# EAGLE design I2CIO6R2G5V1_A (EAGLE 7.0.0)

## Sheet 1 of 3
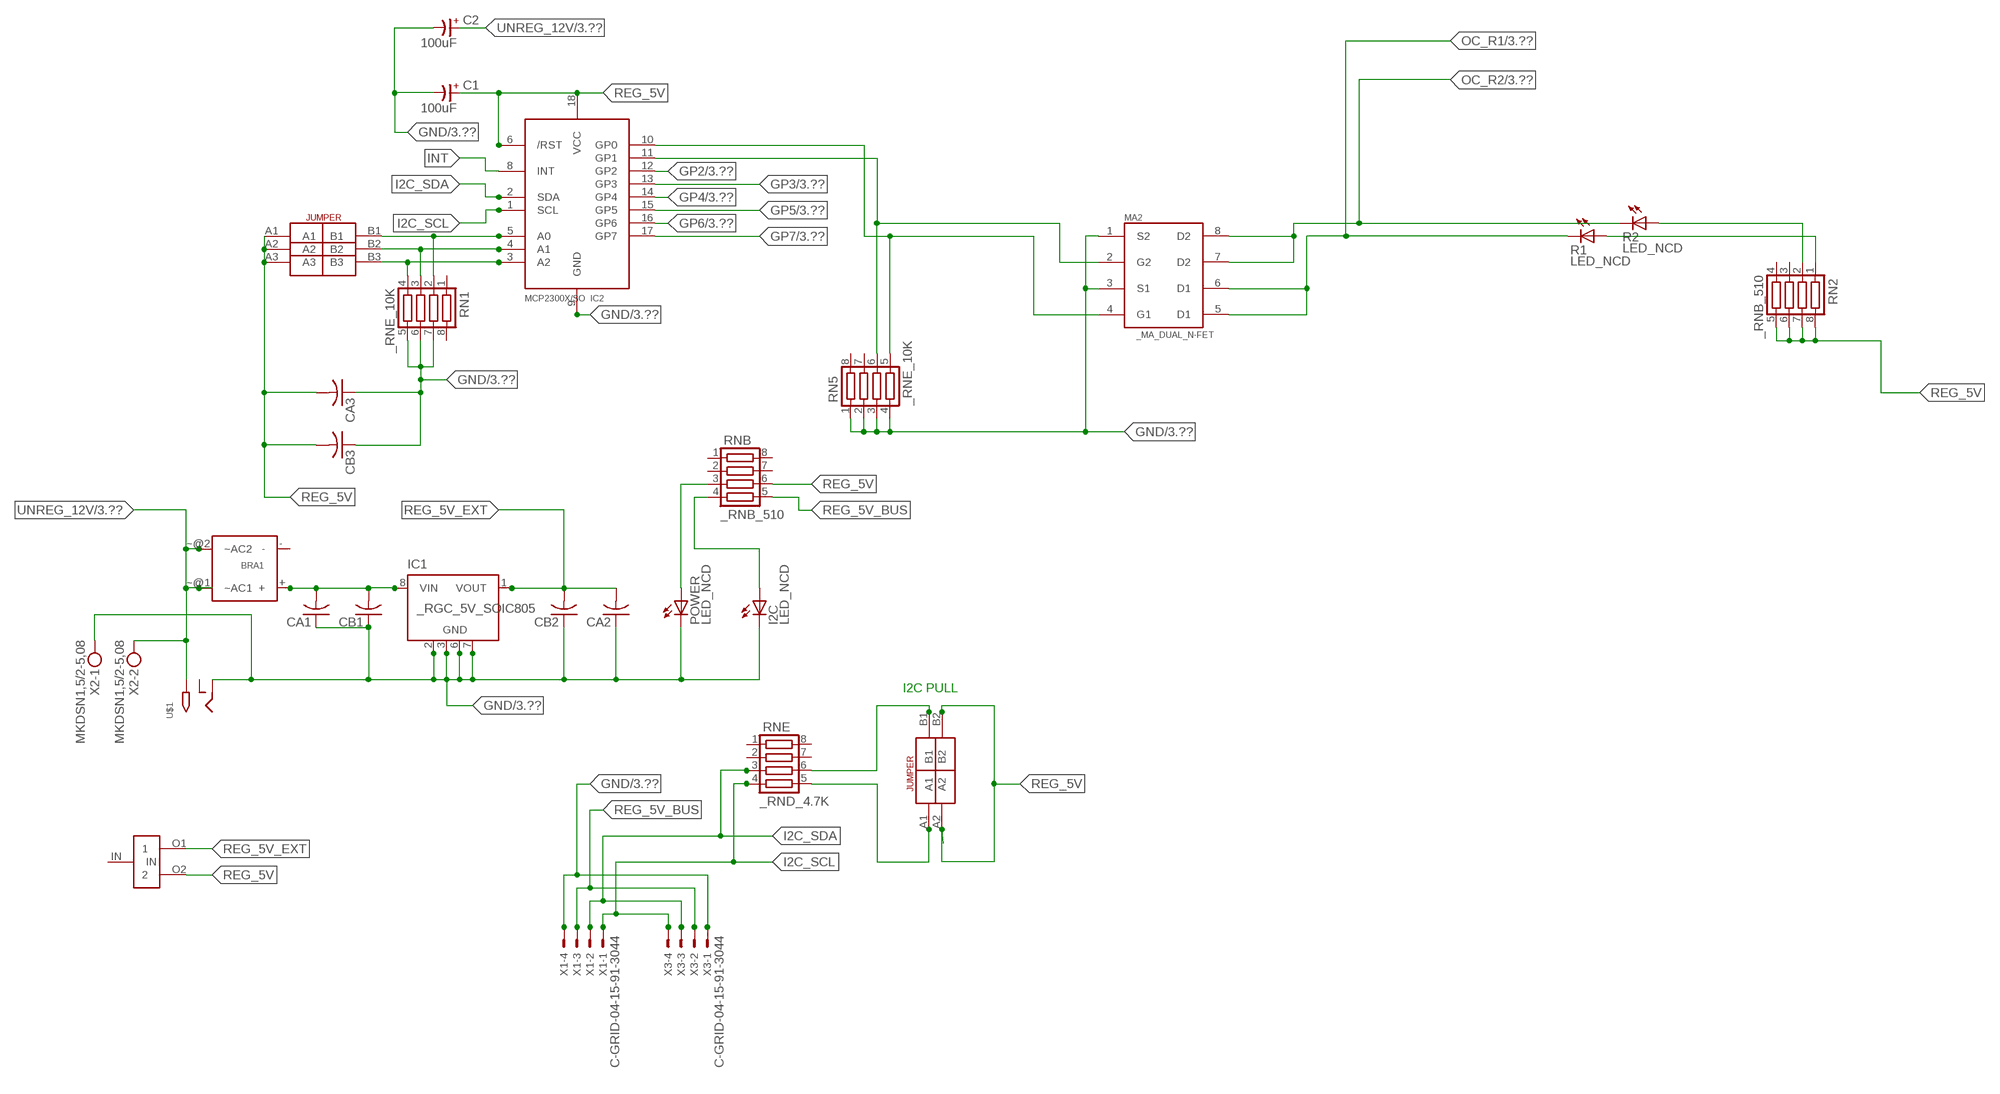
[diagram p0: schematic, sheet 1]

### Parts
BRA1  MB2S_  [MB2S]
C1  100uF  CP-E-025X060  [E-025X060]
C2  100uF  CP-E-025X060  [E-025X060]
CA1  CC1206KRX7R9BB104C1206K  [CC1206KRX7R9BB104]
CA2  CC1206KRX7R9BB104C1206K  [CC1206KRX7R9BB104]
CA3  CC1206KRX7R9BB104C1206K  [CC1206KRX7R9BB104]
CB1  TMK316F106ZL-TC1206K  [TMK316F106ZL-T]
CB2  TMK316F106ZL-TC1206K  [TMK316F106ZL-T]
CB3  TMK316F106ZL-TC1206K  [TMK316F106ZL-T]
I2C  LED_NCD  [CHIPLED_0603]
IC1  _RGC_5V_SOIC805  [_RGC_5V_SOIC8]
IC2  MCP2300X/SO  [SO18W]
MA2  _MA_DUAL_N-FET  [_MA_DUAL_N-FET]
POWER  LED_NCD  [CHIPLED_0603]
R1  LED_NCD  [CHIPLED_0603]
R2  LED_NCD  [CHIPLED_0603]
RN1  _RNE_10K  [RNE]
RN2  _RNB_510  [RNB]
RN5  _RNE_10K  [RNE]
RNB  _RNB_510  [RNB]
RNE  _RND_4.7K  [RND]
U$1  2.1MMJACK  [PJ-102A]
U$3  JUMPER_2X2  [JUMPER_2X2]
U$5  LINK_2  [LINK_2]
U$18  JUMPER_3X2  [JUMPER_3X2]
X1  C-GRID-04-15-91-3044  [15-91-04]
X2  MKDSN1,5/2-5,08  [MKDSN1,5/2-5,08]
X3  C-GRID-04-15-91-3044  [15-91-04]

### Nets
GND: C1.- C2.- CA1.1 CA2.1 CA3.1 CB1.1 CB2.1 CB3.1 I2C.C IC1.2(GND) IC1.3(GND) IC1.6(GND) IC1.7(GND) IC2.9(GND) MA2.1(S2) MA2.3(S1) POWER.C RN1.5 RN1.6 RN1.7 RN5.1 RN5.2 RN5.3 RN5.4 U$1.RING X1.4 X2.1 X3.1 ; also sheet 3
GP2: IC2.12(GP2) ; also sheet 3
GP3: IC2.13(GP3) ; also sheet 3
GP4: IC2.14(GP4) ; also sheet 3
GP5: IC2.15(GP5) ; also sheet 3
GP6: IC2.16(GP6) ; also sheet 3
GP7: IC2.17(GP7) ; also sheet 3
I2C_SCL: IC2.1(SCL) RNE.4 X1.1 X3.4
I2C_SDA: IC2.2(SDA) RNE.3 X1.2 X3.3
INT: IC2.8(INT)
N$1: BRA1.+ CA1.2 CB1.2 IC1.8(VIN)
N$2: POWER.A RNB.3
N$3: I2C.A RNB.4
N$4: RNE.5 U$3.A1
N$5: RNE.6 U$3.B1
N$6: IC2.5(A0) RN1.2 U$18.B1
N$7: IC2.4(A1) RN1.3 U$18.B2
N$8: IC2.3(A2) RN1.4 U$18.B3
N$22: IC2.11(GP1) MA2.2(G2) RN5.6
N$23: IC2.10(GP0) MA2.4(G1) RN5.5
N$31: R2.A RN2.2
N$32: R1.A RN2.1
OC_R1: MA2.5(D1) MA2.6(D1) R1.C ; also sheet 3
OC_R2: MA2.7(D2) MA2.8(D2) R2.C ; also sheet 3
REG_5V: C1.+ CA3.2 CB3.2 IC2.6(/RST) IC2.18(VCC) RN2.5 RN2.6 RN2.7 RN2.8 RNB.6 U$3.A2 U$3.B2 U$5.O2 U$18.A1 U$18.A2 U$18.A3
REG_5V_BUS: RNB.5 X1.3 X3.2
REG_5V_EXT: CA2.2 CB2.2 IC1.1(VOUT) U$5.O1
UNREG_12V: BRA1.~@1(~AC1) BRA1.~@2(~AC2) C2.+ U$1.TIP X2.2 ; also sheet 3
Unconnected: BRA1.- IC1.4(NC) IC1.5(NC) RN1.1 RN1.8 RN2.3 RN2.4 RN5.7 RN5.8 RNB.1 RNB.2 RNB.7 RNB.8 RNE.1 RNE.2 RNE.7 RNE.8 U$1.RING_SW U$5.IN

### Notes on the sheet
- I2C PULL

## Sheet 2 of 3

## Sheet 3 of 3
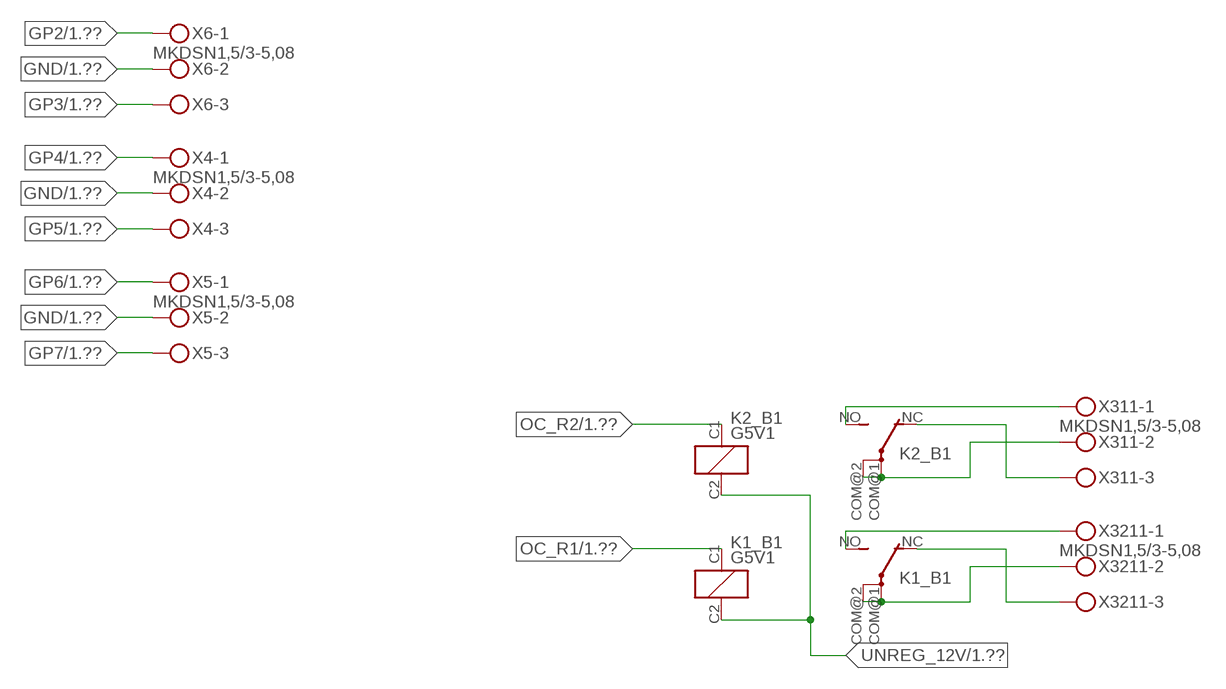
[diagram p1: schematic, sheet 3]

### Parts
K1_B1  G5V1  [G5V1]
K2_B1  G5V1  [G5V1]
X4  MKDSN1,5/3-5,08  [MKDSN1,5/3-5,08]
X5  MKDSN1,5/3-5,08  [MKDSN1,5/3-5,08]
X6  MKDSN1,5/3-5,08  [MKDSN1,5/3-5,08]
X311  MKDSN1,5/3-5,08  [MKDSN1,5/3-5,08]
X3211  MKDSN1,5/3-5,08  [MKDSN1,5/3-5,08]

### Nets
GND: X4.2 X5.2 X6.2 ; also sheet 1
GP2: X6.1 ; also sheet 1
GP3: X6.3 ; also sheet 1
GP4: X4.1 ; also sheet 1
GP5: X4.3 ; also sheet 1
GP6: X5.1 ; also sheet 1
GP7: X5.3 ; also sheet 1
N$221: K2_B1.NO(2:S) X311.1
N$222: K2_B1.NC(2:O) X311.3
N$223: K2_B1.COM@1(2:P) K2_B1.COM@2(2:P) X311.2
N$224: K1_B1.NO(2:S) X3211.1
N$225: K1_B1.NC(2:O) X3211.3
N$226: K1_B1.COM@1(2:P) K1_B1.COM@2(2:P) X3211.2
OC_R1: K1_B1.C1(1:C1) ; also sheet 1
OC_R2: K2_B1.C1(1:C1) ; also sheet 1
UNREG_12V: K1_B1.C2(1:C2) K2_B1.C2(1:C2) ; also sheet 1

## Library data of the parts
BRA1 = NCD_ULTIMATE_LIBRARY:MB2S: Bridge Rectifier BRA MB2S 200V 500ma Digikey MB2S-TPMSTR-ND/MB2S-TP
C1 C2 = NCD_ULTIMATE_LIBRARY:CP-: Capacitors All Kinds POLARIZED CAP
CA1-CA3 = NCD_ULTIMATE_LIBRARY:CC1206KRX7R9BB104: Capacitor CA .1uF 50V SMT C1206K CC1206KRX7R9BB104
CB1-CB3 = NCD_ULTIMATE_LIBRARY:TMK316F106ZL-T: Capacitor CB 10uF SMT 1206 TMK316F106ZL-T
I2C POWER = NCD_ULTIMATE_bhaskar:LED_NCD
IC1 = NCD_ULTIMATE_LIBRARY:_RGC_5V_SOIC8: Regulator Linear 5V Chip Positive VOLTAGE REGULATOR Digikey 497-7267-2-ND/L78L05CD13TR
IC2 = NCD_ULTIMATE_LIBRARY:MCP2300X: Semiconductor Port Expander I/O 8-Bit I2C MCP23008 Inexpensive i2c i/o expander - 8 general purpose i/o pins with optional pullups
K1_B1 K2_B1 = NCD_ULTIMATE_LIBRARY:G5V1: RELAY 1 x switch, 0.5 A/125 V AC, 1 A/24 V DC , Omron
MA2 = NCD_ULTIMATE_LIBRARY:_MA_DUAL_N-FET: FET Dual N-Channel 8-SOIC NMOSFET Digikey 785-1064-2-ND/AO4842
R1 R2 = NCD_ULTIMATE_LIBRARY:LED_NCD: LED Digikey 754-1132-2-ND/APT2012SRCPRV
RN1 RN5 = NCD_ULTIMATE_LIBRARY:_RNE_10K: Resistor Array RNE SMT 10K x 4 Single Resistor Source: http://www.ctscorp.com/components/Datasheets/CTSChipArrayDs.pdf Digikey 742C083103JPTR-ND/742C083103JP; OC_FARNELL: unknown; OC_NEWARK: unknown
RN2 RNB = NCD_ULTIMATE_LIBRARY:_RNB_510: Resistor Array RNB SMT 510 x 4 Single Resistor Source: http://www.ctscorp.com/components/Datasheets/CTSChipArrayDs.pdf Digikey 742C083511JPTR-ND/ 742C083511JP; OC_FARNELL: unknown; OC_NEWARK: unknown
RNE = NCD_ULTIMATE_LIBRARY:_RND_4.7K: Resistor Array RND SMT 4.7K x 4 Single Resistor Source: http://www.ctscorp.com/components/Datasheets/CTSChipArrayDs.pdf Digikey 742C083472JPTR-ND/742C083472JP; OC_FARNELL: unknown; OC_NEWARK: unknown
U$1 = NCD_ULTIMATE_CONNECTORS:2.1MMJACK: 2.1mm x 5.5mm DC jack with internal switch. Digikey part #PJ-102A, 4UCON part #05537 By microbuilder.eu
U$3 = NCD_ULTIMATE_CONNECTORS:JUMPER_2X2
U$5 = NCD_ULTIMATE_LIBRARY:LINK_2: PAD_top
U$18 = NCD_ULTIMATE_CONNECTORS:JUMPER_3X2
X1 X3 = NCD_ULTIMATE_CONNECTORS:C-GRID-04: CONNECTOR 4-Pos I2C wire to board 2.54 mm (0.100") pitch header Digikey WM1342-ND/0015912045; OC_FARNELL: unknown; OC_NEWARK: unknown
X2 = NCD_ULTIMATE_CONNECTORS:MKDSN1,5/2-5,08: MKDSN 1,5/ 2-5,08 Printklemme
X4-X6 X311 X3211 = NCD_ULTIMATE_CONNECTORS:MKDSN1,5/3-5,08: MKDSN 1,5/ 3-5,08 Printklemme Nennstrom: 13,5 A Nennspannung: 250 V Rastermaß: 5,08 mm Polzahl: 3 Anschlussart: Schraubanschluss Montage: Löten Anschlussrichtung Leiter/Platine: 0 ° Artikelnummer: 1729131 Source: http://eshop.phoenixcontact.com .. 1729131.pdf

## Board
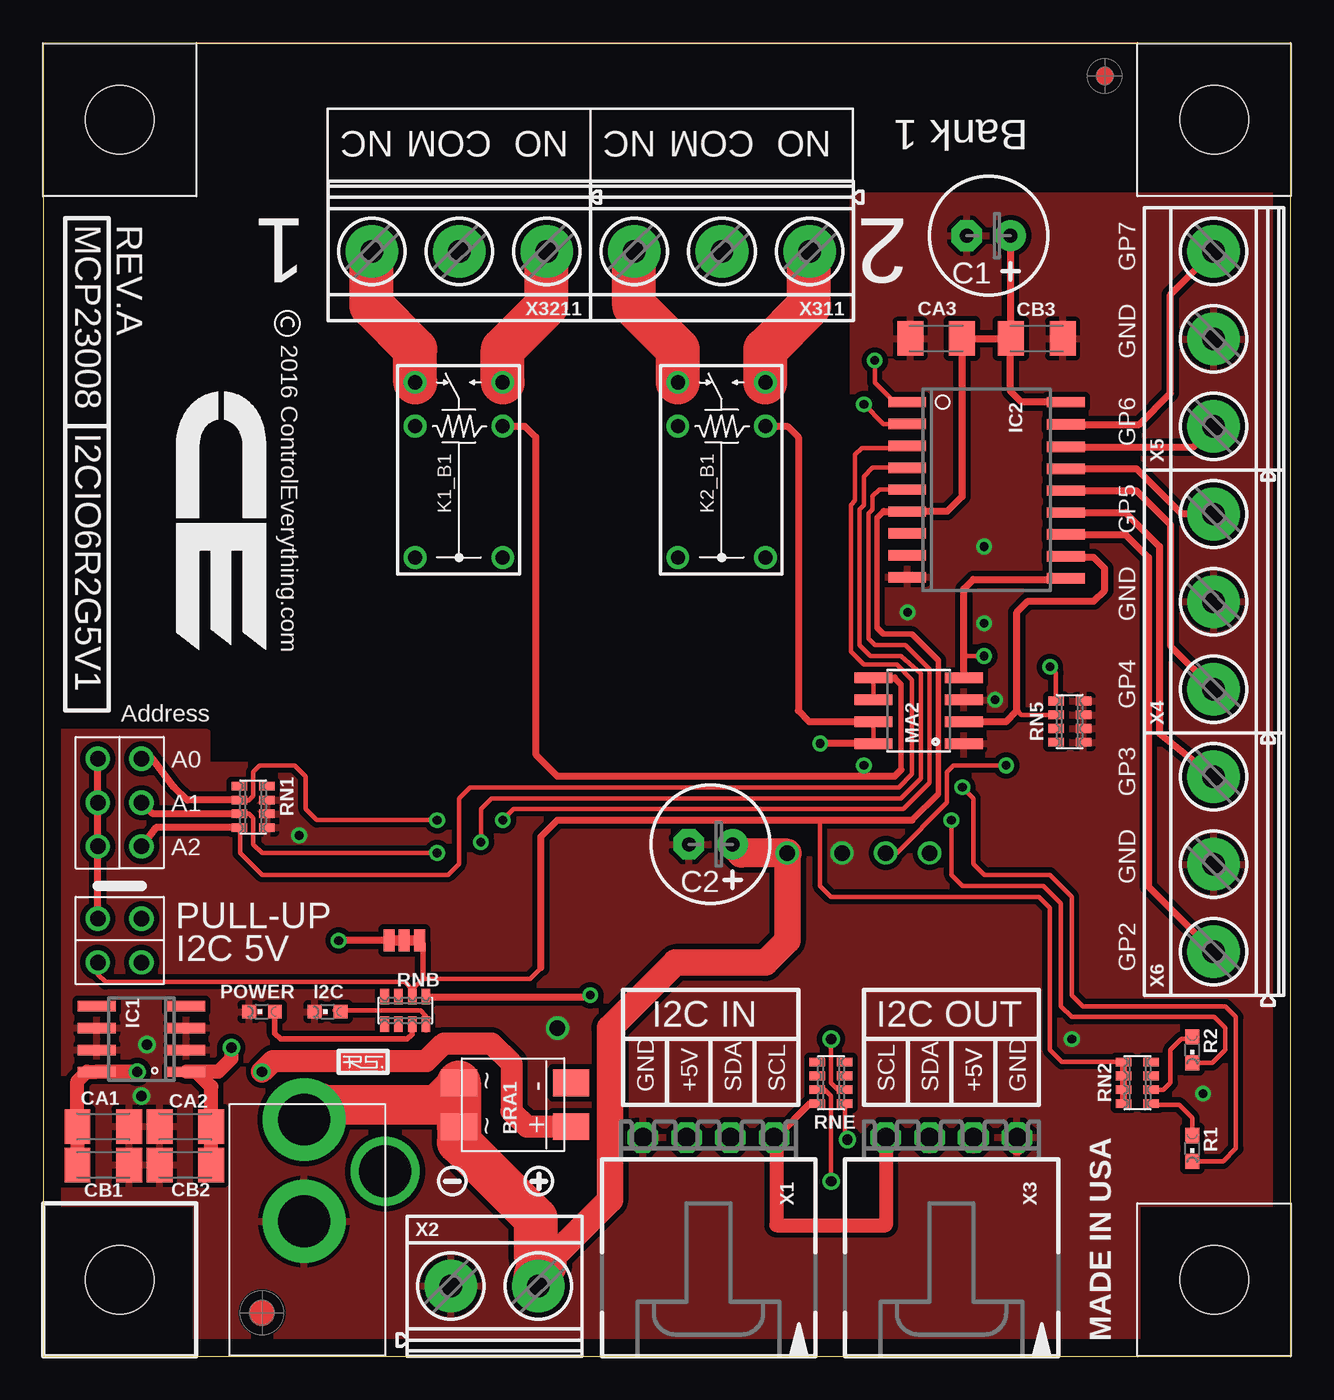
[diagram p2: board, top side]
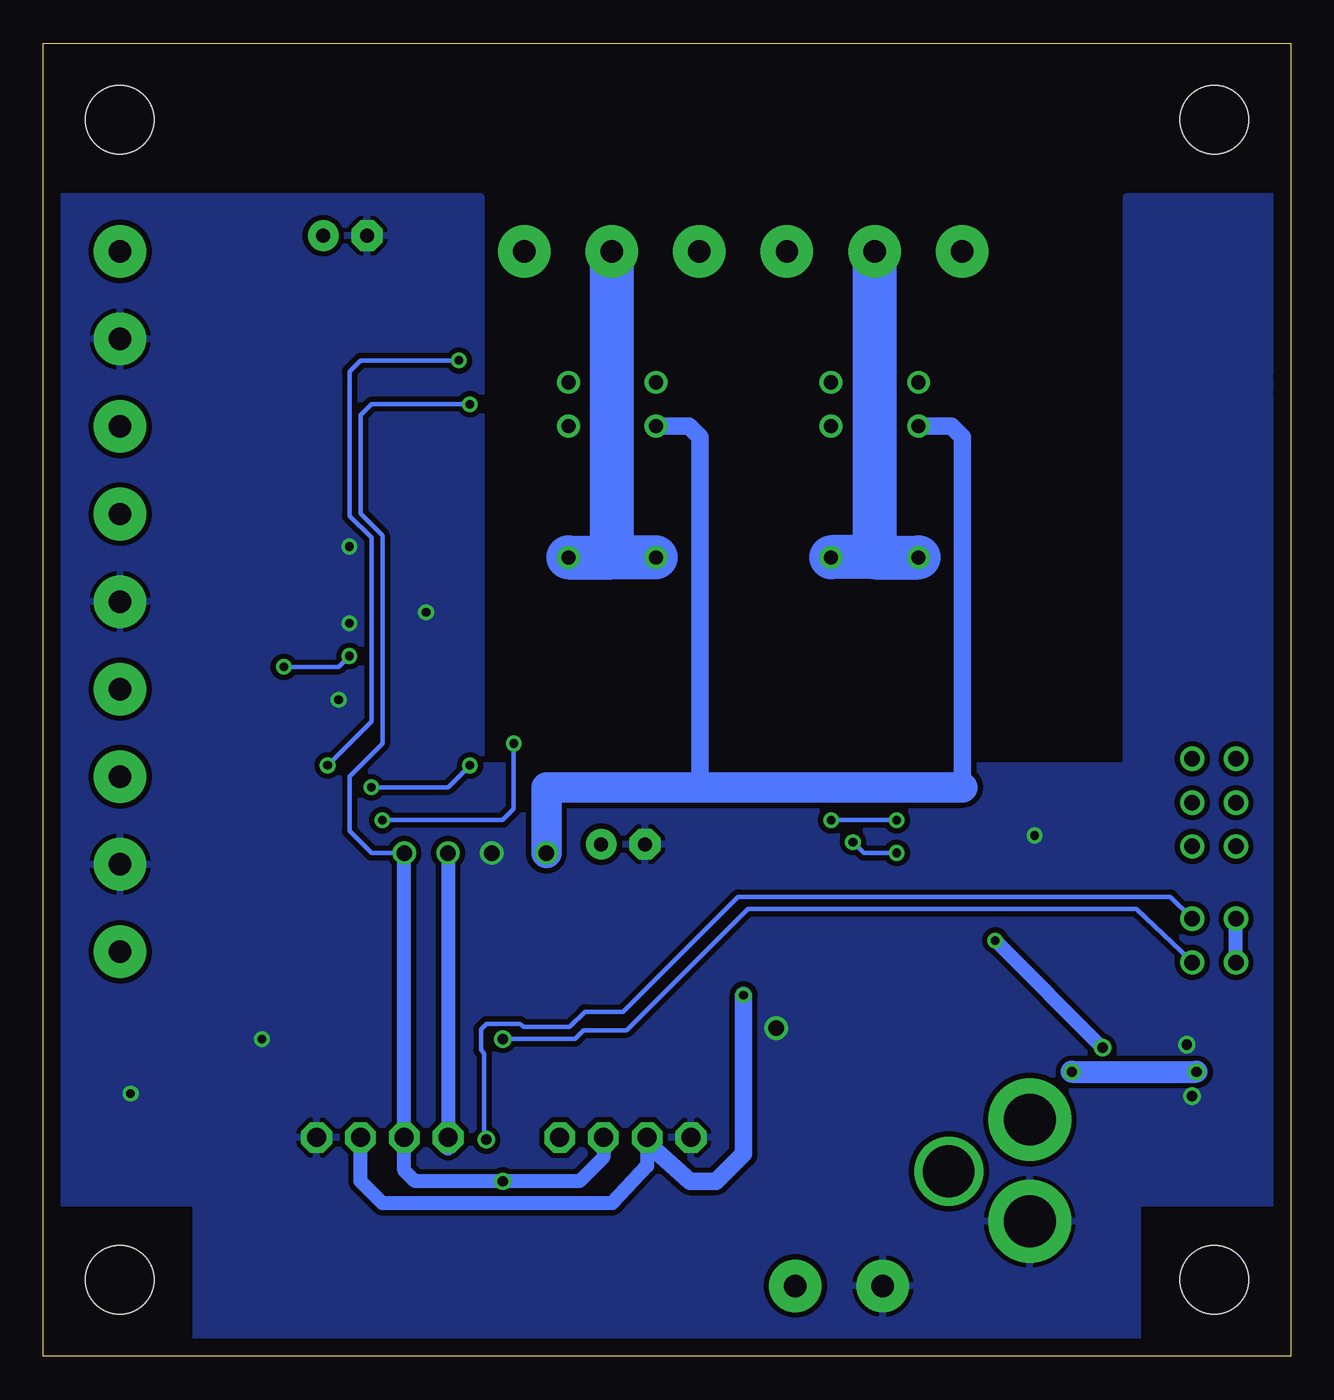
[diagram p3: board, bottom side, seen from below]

Size 72.39 x 76.2 mm. Coordinates in mm from the lower left corner, seen from the top.
Outline: 59.69,0 0,0 0,55.88
Outline: 59.69,0 61.58,0
Outline: 0,56.82 0,55.88
Outline: 59.69,0 72.39,0 72.39,76.2 0,76.2 0,55.88
Copper layers (1*16): Top 0.035mm / dielectric 1.5mm / Bottom 0.035mm
Design rules "default": minimum track width 10mil, minimum drill 24mil, track to track 8mil, track to pad 8mil, pad to pad 8mil, via to via 8mil, smd to smd 8mil, copper to edge 40mil, drill to drill 8mil, minimum pad ring 10mil, minimum via ring 8mil, stop-mask expansion 4mil, vias tented up to drill 0mil, thermal gap 10mil
Holes 3.96 mm at 4.45,4.45

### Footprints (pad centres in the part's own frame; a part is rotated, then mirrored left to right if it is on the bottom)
MB2S = smd 1.55 x 2.1: + 0,-6.5; - 2.54,-6.5; ~@1 0,0; ~@2 2.54,0
E-025X060 = drill 0.813 pad 1.778: + -1.27,0 | drill 0.813 pad 1.778 octagon: - 1.27,0
CC1206KRX7R9BB104 = smd 1.5 x 2: 1 -1.5,0; 2 1.5,0
TMK316F106ZL-T = smd 1.5 x 2: 1 -1.5,0; 2 1.5,0
CHIPLED_0603 = smd 0.8 x 0.8: A 0,-0.75; C 0,0.75
_RGC_5V_SOIC8 = smd 0.6 x 2.2: 1 -1.905,-2.6; 2 -0.635,-2.6; 3 0.635,-2.6; 4 1.905,-2.6; 5 1.905,2.6; 6 0.635,2.6; 7 -0.635,2.6; 8 -1.905,2.6
SO18W = smd 0.6 x 2.2: 1 -4.445,-4.6; 2 -3.175,-4.6; 3 -1.905,-4.6; 4 -0.635,-4.6; 5 0.635,-4.6; 6 1.905,-4.6; 7 3.175,-4.6; 8 4.445,-4.6; 9 5.715,-4.6; 10 5.775,4.6; 11 4.505,4.6; 12 3.235,4.6; 13 1.965,4.6; 14 0.695,4.6; 15 -0.575,4.6; 16 -1.845,4.6; 17 -3.145,4.6; 18 -4.445,4.6
G5V1 = drill 0.813: C1 -2.54,2.54; C2 -2.54,-2.54; COM@1 5.08,-2.54; COM@2 5.08,2.54; NC -5.08,-2.54; NO -5.08,2.54
_MA_DUAL_N-FET = smd 0.61 x 2.21: 1 -1.905,-2.616; 2 -0.635,-2.616; 3 0.635,-2.616; 4 1.905,-2.616; 5 1.905,2.616; 6 0.635,2.616; 7 -0.635,2.616; 8 -1.905,2.616
CHIPLED_0603' = smd 0.8 x 0.876: A 0,-0.75; C 0,0.75
RNE = smd 0.5 x 0.9: 1 -1.2,-0.8; 2 -0.4,-0.8; 3 0.4,-0.8; 4 1.2,-0.8; 5 1.2,0.8; 6 0.4,0.8; 7 -0.4,0.8; 8 -1.2,0.8
RNB = smd 0.5 x 0.9: 1 -1.2,-0.8; 2 -0.4,-0.8; 3 0.4,-0.8; 4 1.2,-0.8; 5 1.2,0.8; 6 0.4,0.8; 7 -0.4,0.8; 8 -1.2,0.8
RND = smd 0.5 x 0.9: 1 -1.2,-0.8; 2 -0.4,-0.8; 3 0.4,-0.8; 4 1.2,-0.8; 5 1.2,0.8; 6 0.4,0.8; 7 -0.4,0.8; 8 -1.2,0.8
PJ-102A = drill 3 pad 4.8: RING 0.1,-3.39; TIP 0.1,-9.29 | drill 3 pad 3.251: RING_SW -4.6,-6.29
JUMPER_2X2 = drill 0.9: A1 0,2.54; A2 0,0; B1 2.54,2.54; B2 2.54,0
PCB_MOUNTING_HOLE = hole 3.962: 4.445,4.445
LINK_2 = smd 1.27 x 0.635: IN 0,0; O1 0,0.889; O2 0,-0.889
JUMPER_3X2 = drill 0.9: A1 0,5.08; A2 0,2.54; A3 0,0; B1 2.54,5.08; B2 2.54,2.54; B3 2.54,0
15-91-04 = drill 1.1 pad 1.778 octagon: 1 -3.81,-7.62; 2 -1.27,-7.62; 3 1.27,-7.62; 4 3.81,-7.62
MKDSN1,5/2-5,08 = drill 1.3 pad 3.048: 1 -2.561,0.025; 2 2.519,0.025
MKDSN1,5/3-5,08 = drill 1.3 pad 3.048: 1 -7.641,0.025; 2 -2.561,0.025; 3 2.519,0.025

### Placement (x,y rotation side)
BRA1  24.13,13.34 90 top
C1  54.86,65.02 180 top
C2  38.73,29.72 180 top
CA1  3.49,13.34 180 top
CA2  8.26,13.34 0 top
CA3  51.82,59.05 0 top
CB1  3.49,11.11 180 top
CB2  8.26,11.11 0 top
CB3  57.66,59.05 180 top
I2C  16.51,20 90 top
IC1  5.71,18.41 90 top
IC2  54.74,50.93 270 top
K1_B1  24.13,51.44 270 top
K2_B1  39.37,51.44 270 top
MA2  50.8,37.47 90 top
POWER  12.7,20 90 top
R1  LED_NCD  [CHIPLED_0603']  66.67,12.06 180 top
R2  LED_NCD  [CHIPLED_0603']  66.67,17.78 180 top
RN1  12.19,31.88 270 top
RN2  63.5,15.88 90 top
RN5  59.56,36.83 90 top
RNB  21.02,20.07 0 top
RNE  45.72,15.88 270 top
U$1  15.24,4.45 180 top
U$3  3.17,25.4 270 top
U$4  PCB_MOUNTING_HOLE  [PCB_MOUNTING_HOLE]  72.39,67.31 90 top
U$5  20.95,24.13 90 top
U$6  PCB_MOUNTING_HOLE  [PCB_MOUNTING_HOLE]  72.39,0 90 top
U$10  [VISION_REF15]  12.7,2.54 0 top
U$11  PCB_MOUNTING_HOLE  [PCB_MOUNTING_HOLE]  8.89,67.31 90 top
U$18  3.17,29.59 0 top
U$19  [VISION_REF10]  61.59,74.3 0 top
U$21  [ICON_USA]  61.98,0.89 90 top
U$22  [ICON_MINUS]  23.75,10.16 180 top
U$24  [ICON_PLUS]  28.77,10.16 90 top
X1  38.61,5.08 180 top
X2  26.23,4.06 0 top
X3  52.7,5.08 180 top
X4  67.94,46.35 90 top
X5  67.94,61.59 90 top
X6  67.94,31.11 90 top
X311  36.83,64.14 180 top
X3211  21.59,64.14 180 top

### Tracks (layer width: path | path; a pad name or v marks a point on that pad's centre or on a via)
GND  (via drill 0.5, 0.6, 0.9)
  Top 0.406: 34.8,12.38 X1.4
  Top 0.813: X3.1 56.52,12.06
  other vias: 5.71,15.11 6.03,18.1 46.35,29.21 29.84,19.05 14.86,30.23 54.61,42.55 54.61,46.99 59.69,18.41 67.31,15.24 50.16,43.18 55.24,38.1
  pour Bottom (isolate 0.305): 0.64,8.89 8.89,8.89 8.89,0 63.5,0 63.5,8.89 71.75,8.89 71.75,67.31 46.99,67.31 46.99,34.29 9.53,34.29 9.53,67.31 0.64,67.31
  pour Top (isolate 0.305): -1.27,8.89 8.89,8.89 8.89,0 63.5,0 63.5,8.89 71.75,8.89 71.75,67.31 46.99,67.31 46.99,34.29 9.53,34.29 9.53,36.2 -1.27,36.2
GP2
  Top 0.406: IC2.12 62.8,47.69 64.14,46.35 64.14,27.26 X6.1
GP3
  Top 0.406: IC2.13 62.8,48.96 64.77,46.99 64.77,36.15 X6.3
GP4
  Top 0.406: IC2.14 63.43,50.23 65.41,48.26 65.41,41.23 X4.1
GP5
  Top 0.406: IC2.15 63.43,51.5 66.04,48.9 67.9,48.9 X4.3
GP6
  Top 0.406: IC2.16 66.74,52.77 X5.1
GP7
  Top 0.406: IC2.17 63.6,54.07 65.41,55.88 65.41,61.6 X5.3
I2C_SCL  (via drill 0.5, 0.9)
  Top 0.254: IC2.1 49.4,55.37 48.26,56.52 v48.26,57.78 | v55.88,34.29 52.83,34.29 52.45,33.91 52.45,32.13 49.53,29.21 v48.9,29.21
  Top 0.406: RNE.4 44.51,14.68 42.55,12.7
  Top 0.813: X3.4 48.9,7.62 42.55,7.62 42.55,12.7 X1.1
  Bottom 0.254: v48.26,57.78 53.98,57.78 54.61,57.15 54.61,48.77 53.34,47.5 53.34,36.83 v55.88,34.29
  Bottom 0.813: v48.9,29.21 X3.4 48.9,12.06
I2C_SDA  (via drill 0.5, 0.6, 0.9)
  Top 0.254: RNE.3 45.36,15.47 45.72,15.11 v45.72,10.16 | IC2.2 48.77,54.1 v47.62,55.24
  Top 0.61: X3.3 51.44,12.06 | X1.2 39.88,12.38
  Bottom 0.254: v47.62,55.24 53.34,55.24 53.98,54.61 53.98,48.9 52.7,47.62 52.7,35.56 54.61,33.66 54.61,30.48 53.34,29.21 v51.44,29.21
  Bottom 0.406: 39.88,12.38 X1.2
  Bottom 0.813: 39.88,12.38 39.88,11.56 41.27,10.16 v45.72,10.16 50.8,10.16 51.44,10.79 X3.3 v51.44,29.21
N$1  (via drill 0.6)
  Top 0.813: CB1.2 CA1.2 1.99,15.96 2.54,16.51 IC1.8 v5.46,16.51
  Top 1.27: v12.7,16.51 13.34,17.14 22.23,17.14 23.24,18.16 26.04,18.16 27.18,17.02 27.18,14.22 28.07,13.34 BRA1.+
  Bottom 1.27: v12.7,16.51 v5.46,16.51
N$2
  Top 0.305: RNB.3 21.4,18.95 21.4,18.7 21.12,18.41 13.78,18.41 13.45,18.74 POWER.A
N$3
  Top 0.254: 22.23,18.95 22.23,19.74 21.9,20.07 16.94,20.07
  Top 0.305: RNB.4 22.23,18.95 | 16.94,20.07 I2C.A
N$4  (via drill 0.6)
  Top 0.254: RNE.5 46.52,12.6 v46.67,12.57
  Bottom 0.254: U$3.A1 6.99,26.67 32.07,26.67 38.73,20 40.96,20 41.85,19.11 44.51,19.11 44.7,19.3 46.67,19.3 46.99,18.99 46.99,17.78 46.8,17.59 46.8,12.7 v46.67,12.57
N$5  (via drill 0.6)
  Top 0.254: RNE.6 46.12,15.47 45.72,15.88 v45.72,18.41
  Bottom 0.254: v45.72,18.41 41.53,18.41 41.02,18.92 38.54,18.92 31.5,25.97 8.95,25.97 6.35,23.5 U$3.B1
N$6  (via drill 0.5)
  Top 0.254: v26.67,31.11 27.3,31.75 49.91,31.75 51.44,33.27 51.44,39.88 50.04,41.27 48.26,41.27 47.88,41.66 47.88,48.9 48.13,49.15 48.13,49.91 48.51,50.29 IC2.5 50.01,50.16 | v22.86,31.11 15.88,31.11 15.24,31.75 15.24,33.66 14.61,34.29 12.57,34.29 12.19,33.91 12.19,32.51 11.94,32.26 11.41,32.26 RN1.2
  Top 0.406: RN1.2 8.36,32.28 7.62,33.02 6.35,34.67 U$18.B1
  Bottom 0.254: v26.67,31.11 v22.86,31.11
N$7  (via drill 0.5)
  Top 0.254: v25.4,29.84 25.4,31.75 26.04,32.38 49.78,32.38 50.93,33.53 50.93,39.62 49.78,40.64 48.01,40.64 47.37,41.27 47.37,49.15 47.62,49.4 47.62,51.05 48.13,51.56 IC2.4 50.01,51.44 | v22.86,29.21 12.7,29.21 12.19,29.72 12.19,31.24 11.94,31.5 11.41,31.5 RN1.3
  Top 0.406: RN1.3 6.37,31.48 U$18.B2
  Bottom 0.254: v25.4,29.84 24.77,29.21 v22.86,29.21
N$8
  Top 0.254: RN1.4 11.43,30.64 11.43,29.21 12.7,27.94 23.5,27.94 24.13,28.57 24.13,32.38 24.77,33.02 49.66,33.02 50.42,33.78 50.42,39.24 49.53,40.13 47.62,40.13 46.86,40.89 46.86,49.4 47.12,49.66 47.12,52.32 47.5,52.7 50.01,52.7 IC2.3
  Top 0.406: RN1.4 6.53,30.68 U$18.B3
N$22
  Top 0.254: RN5.6 56.75,37.23 56.52,37.47
  Top 0.406: MA2.2 55.88,36.83 56.52,37.47 56.52,43.18 57.15,43.81 60.96,43.81 61.59,44.45 61.59,45.72 60.96,46.35 59.4,46.35 IC2.11
N$23  (via drill 0.5)
  Top 0.254: RN5.5 58.76,39.66 v58.42,40.01 | v54.61,40.64 53.42,40.64
  Top 0.406: MA2.4 53.42,40.64 53.42,44.53 53.98,45.09 59.27,45.09 IC2.10
  Bottom 0.254: v58.42,40.01 55.24,40.01 v54.61,40.64
N$31
  Top 0.254: RN2.2 65,15.47 65.41,15.88 65.41,17.78 66.04,18.41 66.56,18.41 R2.A
N$32
  Top 0.254: R1.A 66.67,13.84 65.91,14.61 64.37,14.61 RN2.1
N$221
  Top 2.54: K2_B1.NO 41.91,58.42 44.45,60.96 44.45,64.09 X311.1
N$222
  Top 2.54: K2_B1.NC 36.83,58.42 34.29,60.96 34.29,64.09 X311.3
N$223
  Bottom 2.54: K2_B1.COM@1 39.37,46.35 | K2_B1.COM@2 39.37,46.35 | 39.37,46.35 39.37,64.09 X311.2
N$224
  Top 2.54: K1_B1.NO 26.67,58.42 29.21,60.96 29.21,64.09 X3211.1
N$225
  Top 2.54: K1_B1.NC 21.59,58.42 19.05,60.96 19.05,64.09 X3211.3
N$226
  Bottom 2.54: X3211.2 24.15,46.38 | 24.15,46.38 24.13,46.35 K1_B1.COM@1 | 24.15,46.38 26.65,46.38 K1_B1.COM@2
OC_R1  (via drill 0.5)
  Top 0.254: MA2.5 MA2.6 | R1.C 68.47,11.31 69.22,12.06 69.22,19.68 68.58,20.32 60.33,20.32 59.69,20.95 59.69,26.67 58.42,27.94 54.61,27.94 53.98,28.57 53.98,32.38 v53.34,33.02 | v47.62,34.29 47.62,33.66
  Top 0.305: 49.4,39.37 49.78,38.99 49.78,34.04
  Top 0.406: MA2.5 49.4,39.37 | 49.78,34.04 49.4,33.66 47.62,33.66 29.84,33.66 28.57,34.92 28.57,53.34 27.94,53.98 K1_B1.C1
  Bottom 0.254: v53.34,33.02 48.9,33.02 v47.62,34.29
OC_R2  (via drill 0.5)
  Top 0.254: MA2.7 MA2.8 | R2.C 67.83,17.03 68.58,17.78 68.58,19.05 67.94,19.68 59.69,19.68 59.05,20.32 59.05,26.29 58.04,27.3 53.34,27.3 52.7,27.94 v52.7,31.11
  Top 0.406: K2_B1.C1 43.18,53.98 43.81,53.34 43.81,37.47 44.45,36.83 MA2.7 | MA2.8 v45.09,35.56
  Bottom 0.254: v52.7,31.11 45.72,31.11 45.09,31.75 v45.09,35.56
REG_5V
  Top 0.254: RNB.6 21.42,21.29 | 21.42,21.29 22.04,21.91 28.26,21.91 28.89,22.54 | 21.42,21.29 20.99,21.72 3.62,21.72 3.17,22.16 U$3.B2 | RN2.5 59.12,17.07 58.42,17.78 58.42,26.04 57.78,26.67 45.72,26.67 45.09,27.3 45.09,31.11
  Top 0.305: 50.42,31.11 51.94,32.64 51.94,40.39 50.42,41.91 48.77,41.91 48.39,42.29 48.39,48.64 48.77,49.02 | 22.04,21.91 22.04,23.94 U$5.O2
  Top 0.406: U$18.A1 U$18.A2 U$18.A3 U$3.A2 | RN2.8 RN2.7 RN2.6 RN2.5 | 28.89,22.54 28.89,30.16 29.84,31.11 45.09,31.11 50.42,31.11 | 48.77,49.02 IC2.6 52.45,49.02 53.32,49.89 CA3.2 CB3.2 56.13,59.03 | IC2.18 56.77,55.37 56.13,56.01 56.13,59.03 | C1.+ 56.13,59.03
  Bottom 0.813: U$3.B2 U$3.A2
REG_5V_BUS  (via drill 0.5)
  Top 0.406: RNB.5 31.66,20.87 v31.75,20.95
  Top 0.61: X1.3 37.34,12.38 | X3.2 53.98,12.06
  Bottom 0.406: 37.34,12.38 X1.3 | 53.98,12.06 X3.2
  Bottom 0.813: 37.34,12.38 37.34,11.05 39.37,8.89 52.7,8.89 53.98,10.16 53.98,12.06
  Bottom 1.016: 37.34,12.38 34.86,10.16 33.34,10.16 31.75,11.75 v31.75,20.95
REG_5V_EXT  (via drill 0.5, 0.6)
  Top 0.406: U$5.O1 v17.14,24.13
  Top 0.813: CB2.2 CA2.2 9.76,15.64 8.89,16.51 | 8.89,16.51 IC1.1 | v10.92,17.91 10.92,17.27 10.16,16.51 8.89,16.51
  Bottom 0.813: v17.14,24.13 v10.92,17.91
UNREG_12V  (via drill 0.9)
  Top 1.524: v43.18,29.21 43.18,24.13 41.91,22.86 36.7,22.86 32.89,19.05 32.89,9.08 29.11,5.3 28.57,4.76
  Top 1.676: v43.18,29.21 40.51,29.21 C2.+
  Top 2.286: BRA1.~@2 22.86,14.61 16.01,14.61
  Top 2.54: 16.01,14.61 U$1.TIP | X2.2 28.55,4.45 28.57,4.76 | BRA1.~@2 BRA1.~@1 24.13,12.45 28.57,8 28.57,5.84 29.11,5.3
  Bottom 1.016: K1_B1.C2 19.68,53.98 19.05,53.34 19.05,33.02 | K2_B1.C2 34.92,53.98 34.29,53.34 34.29,33.66 33.66,33.02
  Bottom 1.778: v43.18,29.21 43.18,33.02 33.66,33.02 19.05,33.02

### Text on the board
tNames: Bank 1 | NC | COM | NO | NC | COM | NO | MCP23008 | REV.A | 1 | 2 | GP7 | 2016 ControlEverything.com | GND | I2CIO6R2G5V1 | GP6 | GP5 | GND | GP4 | Address | A0 | GP3 | A1 | A2 | GND | PULL-UP | I2C 5V | GP2 | I2C IN | I2C OUT | GND | +5V | SDA | SCL | SCL | SDA | +5V | +5V | GND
